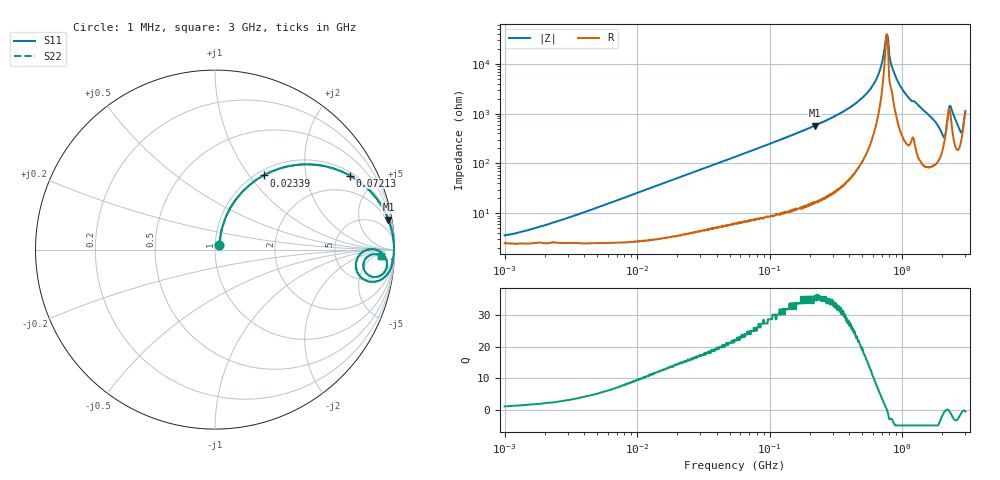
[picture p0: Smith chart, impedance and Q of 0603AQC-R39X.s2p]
!s-Parameter Generated by FASTRON Sdn. Bhd.
!FASTRON P/N : 0603AQC-R39X
!Keysight Technologies: E4991B_MY54100416_A.01.15
!Date: Thu Jun 25 14:08:26 2026
!Version  :Rev00  Thu Jun 25 14:08:26 2026
!Data & Calibration Information:
!Freq  S11  S21  S12  S22
!PortZ  Port1:50+j0  Port2:50+j0
!When reading reference impedance value at option line is always used.
! Remarks : This data is being provided solely for informational purposes.
# Hz S dB R 50
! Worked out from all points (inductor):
!   1601 points, 1 MHz to 3 GHz, reference 50 ohm
!   read as one part in series: L = 408 nH near 2.977 MHz
!   highest Q = 35.8 at 220.1 MHz (marker M1), where L = 417 nH
!   self-resonance near 765.3 MHz
!   S11 on the Smith chart (normalised r, x): 1 MHz: 1.05, +0.05; 23.39 MHz: 1.08, +1.18; 72.13 MHz: 1.14, +3.57; 3 GHz: 21, -10
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1000000  -29.10 44.5  -0.22 -1.4  -0.22 -1.4  -29.10 44.5
3804036  -20.20 70.2  -0.25 -5.4  -0.25 -5.4  -20.20 70.2
1.447069e7  -9.45 65.6  -0.78 -19.6  -0.78 -19.6  -9.45 65.6
2.339465e7  -6.12 56.7  -1.54 -29.6  -1.54 -29.6  -6.12 56.7
5.504702e7  -2.05 35.3  -4.75 -52.1  -4.75 -52.1  -2.05 35.3
7.212514e7  -1.33 28.7  -6.36 -59.0  -6.36 -59.0  -1.33 28.7
2.083556e8  -0.19 10.4  -14.90 -78.0  -14.90 -78.0  -0.19 10.4
2.201458e8  -0.17 9.8  -15.40 -78.6  -15.40 -78.6  -0.17 9.8
3.667557e8  -0.06 5.0  -21.20 -83.1  -21.20 -83.1  -0.06 5.0
5.284703e8  -0.03 2.4  -27.60 -84.2  -27.60 -84.2  -0.03 2.4
6.619339e8  -0.02 0.9  -35.80 -80.0  -35.80 -80.0  -0.02 0.9
7.576891e8  -0.02 0.1  -50.90 -23.5  -50.90 -23.5  -0.02 0.1
7.925923e8  -0.01 -0.3  -46.40 68.8  -46.40 68.8  -0.01 -0.3
8.501091e8  -0.03 -0.7  -37.90 73.7  -37.90 73.7  -0.03 -0.7
9.977393e8  -0.04 -1.8  -30.00 81.6  -30.00 81.6  -0.04 -1.8
1.721456e9  -0.21 -7.4  -17.80 75.7  -17.80 75.7  -0.21 -7.4
2.01032e9  -1.19 -11.7  -12.80 50.4  -12.80 50.4  -1.19 -11.7
2.102926e9  -2.06 -5.3  -12.90 18.8  -12.90 18.8  -2.06 -5.3
2.301132e9  -0.46 -2.5  -23.60 38.0  -23.60 38.0  -0.46 -2.5
2.741597e9  -1.08 -9.8  -14.10 49.2  -14.10 49.2  -1.08 -9.8
2.825159e9  -1.59 -6.7  -14.10 29.1  -14.10 29.1  -1.59 -6.7
3e9  -0.67 -2.2  -21.70 25.5  -21.70 25.5  -0.67 -2.2
